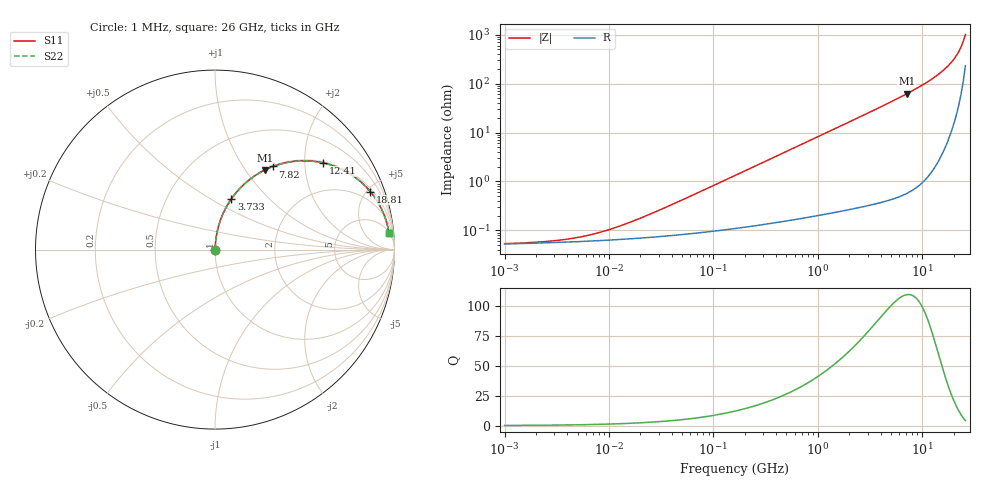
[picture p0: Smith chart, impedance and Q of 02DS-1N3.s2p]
# MHz S MA R 50
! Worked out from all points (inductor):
!   221 points, 1 MHz to 26 GHz, reference 50 ohm
!   read as one part in series: L = 1.3 nH near 27.85 MHz
!   highest Q = 109 at 7.13 GHz (marker M1), where L = 1.38 nH
!   S11 on the Smith chart (normalised r, x): 1 MHz: 1.00, +0.00; 3.733 GHz: 1.01, +0.62; 7.82 GHz: 1.01, +1.38; 12.41 GHz: 1.03, +2.48; 18.81 GHz: 1.19, +5.27; 26 GHz: 6, +20
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1  0.000534 8.8  0.9995 -0.0  0.9995 -0.0  0.000534 8.8
2.63894  0.0005978 21.1  0.9994 -0.0  0.9994 -0.0  0.0005978 21.1
5.52737  0.0007447 37.3  0.9994 -0.0  0.9994 -0.0  0.0007447 37.3
7.9995  0.0008973 46.7  0.9994 -0.0  0.9994 -0.0  0.0008973 46.7
12.1248  0.001182 56.8  0.9994 -0.1  0.9994 -0.1  0.001182 56.8
30.5518  0.002602 73.2  0.9993 -0.1  0.9993 -0.1  0.002602 73.2
168.871  0.01382 84.6  0.9988 -0.8  0.9988 -0.8  0.01382 84.6
425.516  0.03472 85.6  0.9979 -2.0  0.9979 -2.0  0.03472 85.6
891.261  0.07256 84.3  0.9955 -4.2  0.9955 -4.2  0.07256 84.3
1866.78  0.151 80.4  0.986 -8.7  0.986 -8.7  0.151 80.4
3733.49  0.2952 72.2  0.9521 -17.2  0.9521 -17.2  0.2952 72.2
4926.33  0.3814 67.0  0.9206 -22.4  0.9206 -22.4  0.3814 67.0
7129.64  0.5245 57.8  0.8466 -31.6  0.8466 -31.6  0.5245 57.8
7819.95  0.5646 55.1  0.8202 -34.4  0.8202 -34.4  0.5646 55.1
9852.45  0.6693 47.4  0.7364 -42.0  0.7364 -42.0  0.6693 47.4
12413.2  0.7734 38.6  0.6241 -50.7  0.6241 -50.7  0.7734 38.6
15639.6  0.866 28.8  0.4825 -60.0  0.4825 -60.0  0.866 28.8
18814.7  0.9238 20.5  0.3506 -67.4  0.3506 -67.4  0.9238 20.5
20636.4  0.9452 16.2  0.2798 -70.7  0.2798 -70.7  0.9452 16.2
22634.4  0.9611 11.9  0.2069 -73.3  0.2069 -73.3  0.9611 11.9
24825.9  0.9708 7.6  0.133 -73.6  0.133 -73.6  0.9708 7.6
26000  0.9734 5.4  0.09635 -71.3  0.09635 -71.3  0.9734 5.4
